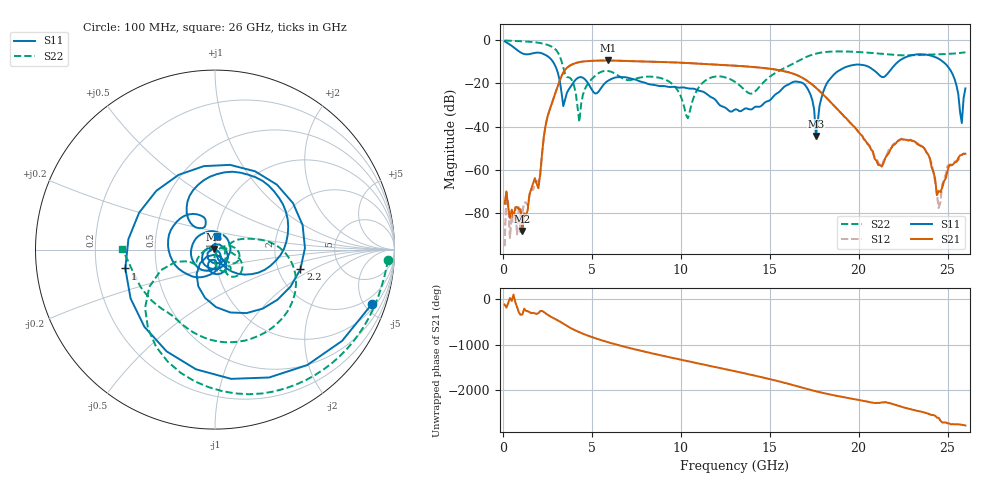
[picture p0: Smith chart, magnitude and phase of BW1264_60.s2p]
!Keysight Technologies,N5245B,MY57181159,A.13.60.06
!Date: Friday, December 18, 2020 23:55:11
!Correction: S11(Full 2 Port(1,2))
!S21(Full 2 Port(1,2))
!S12(Full 2 Port(1,2))
!S22(Full 2 Port(1,2))
!S2P File: Measurements: S11, S21, S12, S22:
# Hz S  dB  R 50
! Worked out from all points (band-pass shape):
!   260 points, 100 MHz to 26 GHz, reference 50 ohm
!   highest |S21| = -9.53 dB at 5.9 GHz (marker M1); lowest = -88.1 dB at 1.1 GHz (marker M2)
!   |S21| within 3 dB of the highest: 3.659 GHz to 14.09 GHz (10.44 GHz wide, 118 % of centre)
!   lowest |S11| = -44.3 dB at 17.6 GHz (marker M3), VSWR 1.01, Z = 49.5 + j0.357 ohm
!   |S11| at or under -10 dB: 2.809 GHz to 22.24 GHz (19.43 GHz wide, 155 % of centre); 24.73 GHz to end of sweep
!   |S22| runs from -37.9 to -0.3 dB; largest |S21 - S12| = 0.00061
!   S11 on the Smith chart (normalised r, x): 100 MHz: 1.33, -5.59; 1 GHz: 0.33, -0.09; 2.2 GHz: 2.65, -0.77; 26 GHz: 1.01, +0.15
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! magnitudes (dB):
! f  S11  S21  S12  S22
! 100 MHz  -0.7  -75.6  -95.1  -0.3
! 1 GHz  -5.8  -78.1  -88.6  -0.6
! 1.1 GHz  -6.3  -88.1  -79.6  -0.7
! 2.2 GHz  -6.2  -52.9  -53.4  -1.6
! 3.4 GHz  -30.6  -15.1  -15.1  -12.9
! 4.3 GHz  -17.3  -10.3  -10.3  -37.9
! 4.5 GHz  -17.5  -10.0  -10.0  -25.4
! 5.9 GHz  -18.9  -9.5  -9.5  -14.3
! 8.8 GHz  -21.3  -10.2  -10.2  -17.5
! 10.4 GHz  -22.4  -10.7  -10.7  -36.2
! 11.4 GHz  -24.6  -11.2  -11.2  -18.7
! 13.1 GHz  -32.0  -11.9  -11.9  -19.6
! 17.4 GHz  -27.9  -20.7  -20.7  -6.8
! 17.6 GHz  -44.3  -22.1  -22.1  -6.4
! 18.7 GHz  -15.3  -31.1  -31.1  -5.4
! 21.3 GHz  -17.1  -58.4  -58.6  -6.5
! 21.7 GHz  -14.9  -52.1  -50.6  -6.8
! 23.6 GHz  -6.7  -49.3  -49.0  -6.9
! 24.5 GHz  -8.7  -69.6  -77.5  -6.7
! 25.4 GHz  -18.3  -56.6  -56.1  -6.3
! 25.8 GHz  -38.4  -53.0  -53.0  -6.0
! 26 GHz  -22.4  -52.5  -52.8  -5.7
